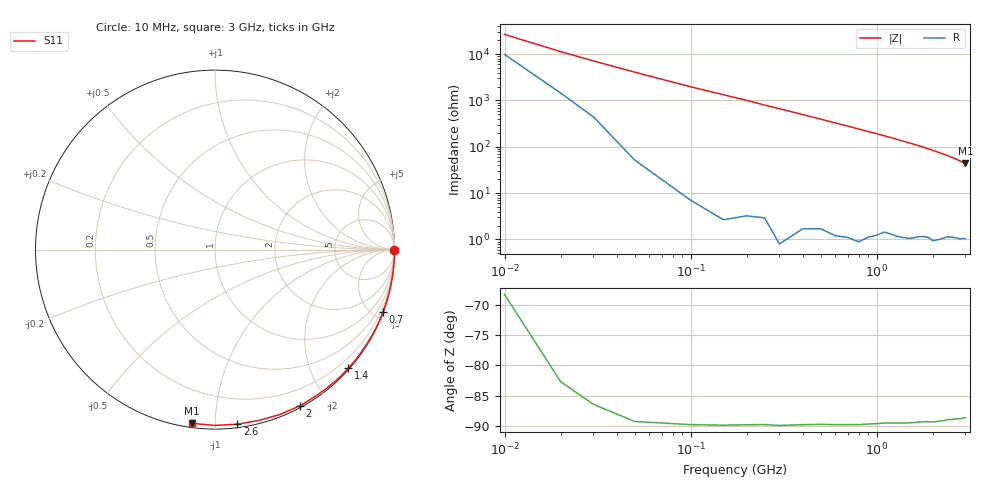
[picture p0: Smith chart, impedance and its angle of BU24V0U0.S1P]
! SIEMENS Small Signal Semiconductors
! BB833
! Si Tuning Diode in SOD323
! VR = 24 V
! S-Parameters:  April  1996
# GHz  S  MA  R  50
!  f  S11
! GHz  MAG  ANG
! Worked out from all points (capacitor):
!   31 points, 10 MHz to 3 GHz, reference 50 ohm
!   read as one part to ground: C = 706 fF near 10 MHz
!   lowest |Z| = 43.7 ohm at 3 GHz (marker M1)
!   S11 on the Smith chart (normalised r, x): 10 MHz: open; 700 MHz: 0.02, -5.59; 1.4 GHz: 0.02, -2.63; 2 GHz: 0.02, -1.68; 2.6 GHz: 0.02, -1.14; 3 GHz: 0.02, -0.87
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0.01  0.9986 -0.2
0.05  0.9997 -1.4
0.1  0.9998 -2.9
0.2  0.9997 -5.7
0.25  0.9995 -7.2
0.3  0.9998 -8.6
0.4  0.9993 -11.5
0.5  0.9989 -14.4
0.6  0.9989 -17.4
0.7  0.9986 -20.3
0.8  0.9986 -23.3
0.9  0.9977 -26.3
1  0.9969 -29.2
1.1  0.9956 -32.3
1.2  0.9952 -35.4
1.3  0.995 -38.5
1.4  0.9944 -41.7
1.5  0.9939 -44.8
1.6  0.9928 -48.0
1.7  0.9914 -51.3
1.8  0.9903 -54.6
1.9  0.9897 -58.0
2  0.9902 -61.4
2.2  0.9873 -68.3
2.4  0.9831 -75.3
2.6  0.9809 -82.7
2.8  0.9795 -90.1
3  0.9767 -97.7
